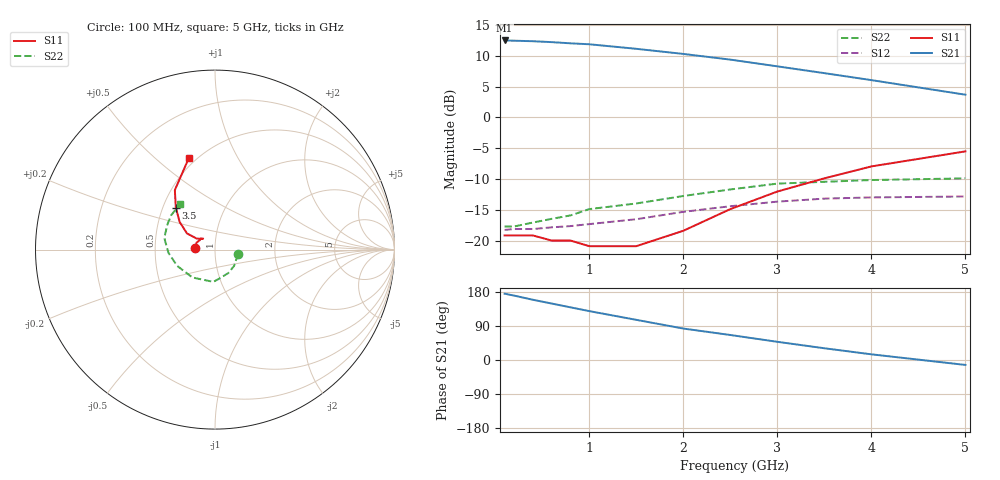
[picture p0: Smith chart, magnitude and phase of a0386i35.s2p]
!  MSA-0386 S AND NOISE PARAMETERS
!  Id=35mA  LAST UPDATED 07-22-92
# ghz s ma r 50
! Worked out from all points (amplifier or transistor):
!   13 points, 100 MHz to 5 GHz, reference 50 ohm
!   highest |S21| = 12.5 dB at 100 MHz (marker M1)
!   |S21| within 3 dB of that: start of sweep to 2.44 GHz
!   unconditionally stable (mu >= 1): start of sweep to end of sweep
!   at 400 MHz: K = 1.19, MAG = 12.6 dB, |S12| = -18.1 dB
!   at 1.5 GHz: K = 1.16, MAG = 11.4 dB, |S12| = -16.5 dB
!   at 5 GHz: K = 1.13, MAG = 6.0 dB, |S12| = -12.8 dB
!   lowest NFmin = 5.60 dB at 100 MHz
!   S11 on the Smith chart (normalised r, x): 100 MHz: 0.80, +0.02; 3.5 GHz: 0.58, +0.30; 5 GHz: 0.46, +0.65
0.1  0.11 174.0  4.22 175.0  0.122 1.0  0.13 -11.0
0.2  0.11 169.0  4.2 170.0  0.124 2.0  0.13 -20.0
0.4  0.11 159.0  4.16 159.0  0.124 5.0  0.14 -41.0
0.6  0.1 149.0  4.09 149.0  0.128 8.0  0.15 -60.0
0.8  0.1 142.0  4 139.0  0.131 9.0  0.16 -78.0
1  0.09 137.0  3.93 129.0  0.136 11.0  0.18 -93.0
1.5  0.09 139.0  3.61 106.0  0.149 14.0  0.2 -129.0
2  0.12 149.0  3.28 83.0  0.171 13.0  0.23 -157.0
2.5  0.18 150.0  2.95 66.0  0.19 12.0  0.26 -176.0
3  0.25 142.0  2.6 48.0  0.207 9.0  0.29 167.0
3.5  0.32 133.0  2.29 31.0  0.219 3.0  0.3 152.0
4  0.4 124.0  2.01 15.0  0.224 -1.0  0.31 142.0
5  0.53 106.0  1.53 -13.0  0.228 -11.0  0.32 128.0
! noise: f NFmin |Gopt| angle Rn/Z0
0.1  5.6  0.05  -1  0.84
0.5  5.8  0.04  -10  0.84
1  6  0.04  -42  0.83
2  6.5  0.07  -91  0.81
